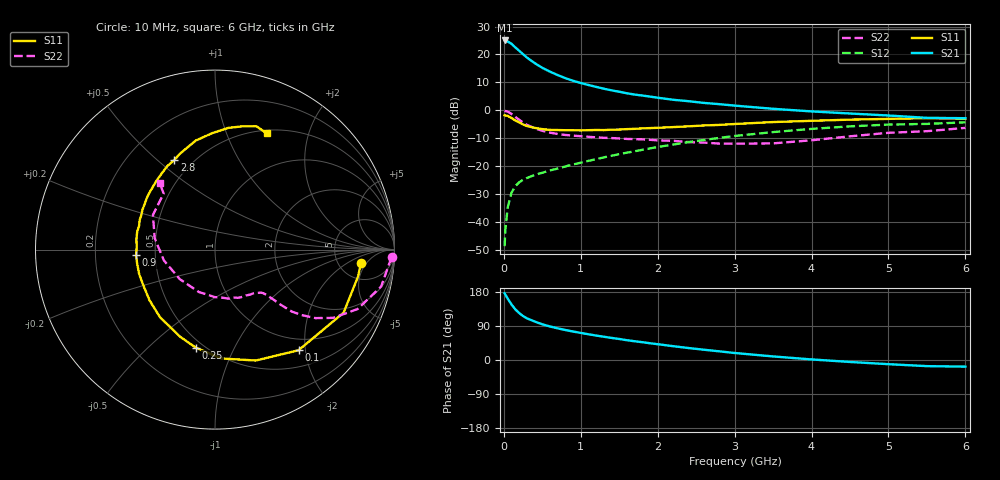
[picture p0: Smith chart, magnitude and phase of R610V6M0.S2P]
! SIEMENS Small Signal Semiconductors
! BFR193
! Si NPN RF Bipolar Junction Transistor in SOT23
! VCE = 10 V  IC = 6 mA
! Common Emitter S-Parameters:  May  1996
# GHz  S  MA  R  50
!  f  S11  S21  S12  S22
! GHz  MAG  ANG  MAG  ANG  MAG  ANG  MAG  ANG
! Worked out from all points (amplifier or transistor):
!   36 points, 10 MHz to 6 GHz, reference 50 ohm
!   highest |S21| = 25.0 dB at 10 MHz (marker M1)
!   |S21| within 3 dB of that: start of sweep to 170.5 MHz
!   unconditionally stable (mu >= 1): 902.3 MHz to 2.052 GHz
!   at 250 MHz: K = 0.47, MSG = 22.5 dB, |S12| = -24.9 dB
!   at 1.4 GHz: K = 1.06, MAG = 10.3 dB, |S12| = -16.3 dB
!   at 6 GHz: K = 0.95, MSG = 0.7 dB, |S12| = -4.3 dB
!   S11 on the Smith chart (normalised r, x): 10 MHz: 8.27, -3.68; 100 MHz: 0.78, -1.87; 250 MHz: 0.45, -0.72; 900 MHz: 0.39, -0.03; 2.8 GHz: 0.40, +0.57; 6 GHz: 0.54, +1.40
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0.01  0.8169 -5.2  17.84 176.3  0.0037 82.5  0.9851 -2.5
0.02  0.8111 -10.6  17.62 172.3  0.0073 81.2  0.9715 -5.1
0.05  0.7981 -26.1  17.07 162.0  0.0183 76.5  0.9486 -12.5
0.1  0.7288 -50.3  15.52 146.4  0.0336 66.7  0.861 -22.6
0.15  0.6585 -69.8  13.35 133.4  0.0441 58.8  0.7608 -30.0
0.2  0.6077 -86.6  11.65 123.8  0.0515 54.6  0.6773 -34.3
0.25  0.5571 -100.9  10.11 115.9  0.0571 51.9  0.6042 -37.1
0.3  0.5238 -111.5  8.827 110.0  0.0616 50.6  0.5496 -38.9
0.4  0.4857 -129.1  7.02 101.5  0.0695 50.0  0.4787 -40.0
0.5  0.4614 -142.2  5.768 94.2  0.0764 50.7  0.4303 -40.5
0.6  0.4465 -153.2  4.928 88.5  0.084 52.3  0.3986 -41.0
0.7  0.444 -162.1  4.282 83.5  0.0906 53.8  0.378 -41.5
0.9  0.4407 -176.0  3.383 75.1  0.1074 55.9  0.3529 -42.9
1.1  0.4415 172.7  2.843 67.9  0.1246 57.9  0.3362 -46.0
1.3  0.4431 162.8  2.44 61.4  0.144 59.1  0.3224 -49.4
1.6  0.4615 151.1  2.02 52.2  0.1748 59.3  0.3079 -56.2
2.2  0.5014 131.1  1.547 36.5  0.244 56.6  0.2846 -74.0
2.8  0.5487 114.3  1.291 22.9  0.3211 50.3  0.2541 -100.1
3.5  0.617 100.0  1.066 9.4  0.408 40.4  0.256 -139.8
4.5  0.6819 83.8  0.878 -5.2  0.5169 24.6  0.3426 169.1
5.5  0.7248 71.5  0.734 -16.2  0.5718 8.0  0.4236 132.5
6  0.7088 65.9  0.723 -17.5  0.6105 3.2  0.4849 129.6
